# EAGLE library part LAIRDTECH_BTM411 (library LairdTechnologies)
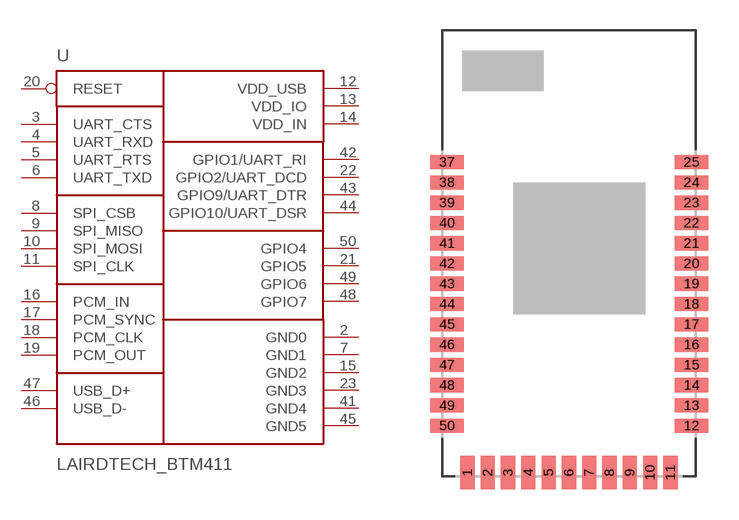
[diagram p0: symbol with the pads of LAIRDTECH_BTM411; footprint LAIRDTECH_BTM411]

Designator prefix -

## LAIRDTECH_BTM411  [LAIRDTECH_BTM411]
2  GND0
3  UART_CTS
4  UART_RXD
5  UART_RTS
6  UART_TXD
7  GND1
8  SPI_CSB
9  SPI_MISO
10  SPI_MOSI
11  SPI_CLK
12  VDD_USB
13  VDD_IO
14  VDD_IN
15  GND2
16  PCM_IN
17  PCM_SYNC
18  PCM_CLK
19  PCM_OUT
20  RESET
21  GPIO5
22  GPIO2/UART_DCD
23  GND3
41  GND4
42  GPIO1/UART_RI
43  GPIO9/UART_DTR
44  GPIO10/UART_DSR
45  GND5
46  USB_D-
47  USB_D+
48  GPIO7
49  GPIO6
50  GPIO4

## Footprint LAIRDTECH_BTM411 (pad centres in mm)
smd 0.7 x 1.65: 1 1.25,0.2; 2 2.25,0.2; 3 3.25,0.2; 4 4.25,0.2; 5 5.25,0.2; 6 6.25,0.2; 7 7.25,0.2; 8 8.25,0.2; 9 9.25,0.2; 10 10.25,0.2; 11 11.25,0.2
smd 1.65 x 0.7: 12 12.3,2.5; 13 12.3,3.5; 14 12.3,4.5; 15 12.3,5.5; 16 12.3,6.5; 17 12.3,7.5; 18 12.3,8.5; 19 12.3,9.5; 20 12.3,10.5; 21 12.3,11.5; 22 12.3,12.5; 23 12.3,13.5; 24 12.3,14.5; 25 12.3,15.5; 37 0.25,15.5; 38 0.25,14.5; 39 0.25,13.5; 40 0.25,12.5; 41 0.25,11.5; 42 0.25,10.5; 43 0.25,9.5; 44 0.25,8.5; 45 0.25,7.5; 46 0.25,6.5; 47 0.25,5.5; 48 0.25,4.5; 49 0.25,3.5; 50 0.25,2.5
